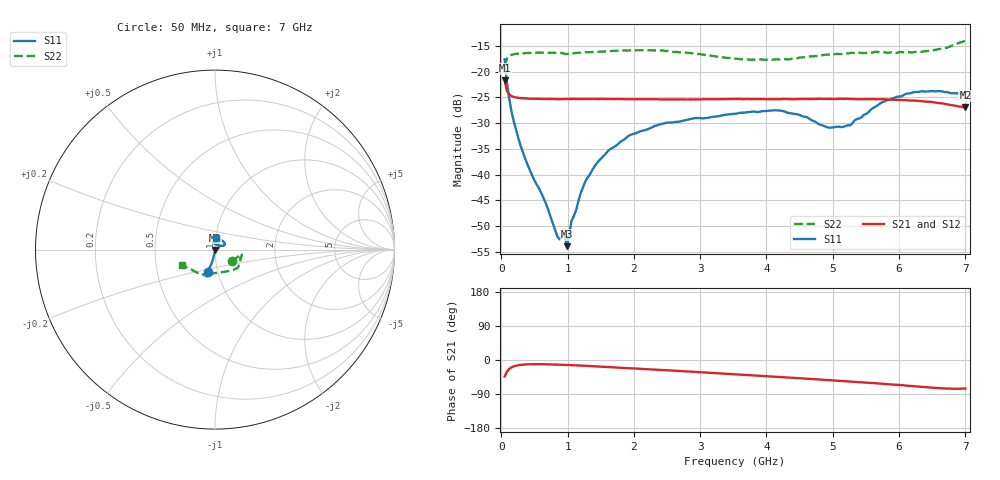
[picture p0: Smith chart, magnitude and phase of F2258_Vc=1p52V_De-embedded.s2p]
! Integrated Device Technology
! Corporate Headquarters
! 6024 Silver Creek Valley Road
! San Jose, CA 95138  USA
! Phone:  1-408-284-8200
! Toll Free:  1-800-223-1366
! Webpage:  http://www.idt.com/
! Timing and RF Division
! 515 Groton Road, Suite 102
! Westford, MA 01886-6024
! Device:  F2258
! Description: Voltage Variable RF Attenuator
! Frequency:  50.0 -  6000.00 MHz
! Package:  3x3 mm Thin QFN Plastic Package: 16 pin
! Ports:  2 RF, 2 DC
!  Pin  1  = NC
!  Pin  2  = NC
!  Pin  3  = RF2  = Port 2
!  Pin  4  = GND
!  Pin  5  = Vdd
!  Pin  6  = NC
!  Pin  7  = VCTRL
!  Pin  8  = NC
!  Pin  9  = GND
!  Pin 10  = RF1  = Port 1
!  Pin 11  = NC
!  Pin 12  = NC
!  Pin 13  = NC
!  Pin 14  = NC
!  Pin 15  = NC
!  Pin 16  = NC
! Vcntrl:  1.520 Volts
! Vdd:  +3.300 Volts
! Current:  1.161 mA
! Data:  The device was measured on a the F2258 evaluation board which has
!  individual transmission lines to the RF pins.  Data was collected
!  using a calibrated network analyzer.  The evaluation board was
!  de-embedded using a TRL calibration technique.
!  The reference plane is the edge of the package pin.
! Misc:  SN 10
!  Action Tracker AT0285
! Date Measured:  2014-12-10
! Date:  2016-01-13  MJV
! Note:
!  Integrated Device Technology supplies this data as a sample of measured
!  data at the package pin for this product.  Your particular data for this
!  product may vary.
!  Data was taken at 25 degrees C.
!  Integrated Device Technology reserves the right to change this data at anytime.
!Freq_(GHz)  S11M_(dB)  S11P_(deg)  S21M_(dB)  S21P_(deg)  S12M_(dB)  S12P_(deg)  S22M_(dB)  S22P_(deg)
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# GHz S dB R 50
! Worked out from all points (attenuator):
!   201 points, 50 MHz to 7 GHz, reference 50 ohm
!   highest |S21| = -21.70 dB at 50 MHz (marker M1); lowest = -26.9 dB at 7 GHz (marker M2)
!   lowest |S11| = -53.9 dB at 988.2 MHz (marker M3), VSWR 1.00, Z = 50.1 - j0.176 ohm
!   |S11| at or under -10 dB: start of sweep to end of sweep
!   |S22| runs from -18.9 to -14.0 dB; largest |S21 - S12| = 0.00055
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0.05  -17.62 -108.5  -21.70 -43.6  -21.68 -43.6  -18.89 -34.7
0.08475  -22.09 -103.7  -23.76 -30.8  -23.69 -30.7  -17.45 -17.1
0.15425  -27.76 -101.1  -24.75 -19.4  -24.71 -19.4  -16.75 -10.5
0.29325  -34.48 -98.7  -25.14 -12.8  -25.11 -12.8  -16.46 -9.0
0.6755  -45.66 -77.9  -25.30 -11.4  -25.28 -11.4  -16.30 -13.3
0.84925  -52.10 -35.2  -25.35 -12.2  -25.31 -12.2  -16.39 -16.4
0.9535  -51.45 -74.7  -25.34 -12.9  -25.31 -12.9  -16.58 -17.8
0.98825  -53.86 -60.1  -25.34 -13.1  -25.28 -13.1  -16.59 -18.8
1.05775  -49.03 -14.0  -25.31 -13.6  -25.30 -13.6  -16.46 -19.8
1.2315  -42.44 10.9  -25.31 -15.0  -25.28 -15.0  -16.28 -22.7
1.40525  -38.42 14.1  -25.30 -16.7  -25.27 -16.7  -16.17 -25.3
1.61375  -35.34 19.1  -25.33 -18.7  -25.28 -18.7  -16.04 -29.0
1.9265  -32.41 27.9  -25.37 -21.7  -25.33 -21.7  -15.89 -33.5
2.37825  -30.28 39.3  -25.40 -26.0  -25.37 -26.0  -15.91 -40.5
3.525  -28.20 87.5  -25.32 -37.7  -25.35 -37.7  -17.47 -68.1
4.1505  -27.50 103.4  -25.35 -44.4  -25.35 -44.4  -17.61 -88.9
4.7065  -29.57 93.5  -25.30 -50.4  -25.31 -50.4  -17.05 -100.5
4.94975  -30.89 76.2  -25.31 -53.1  -25.33 -53.1  -16.71 -103.1
5.2625  -30.43 48.0  -25.33 -56.7  -25.34 -56.7  -16.39 -105.4
5.85325  -25.45 25.7  -25.44 -64.2  -25.44 -64.2  -16.34 -108.9
6.33975  -23.78 32.0  -25.75 -71.0  -25.75 -71.0  -16.16 -120.6
7  -23.95 83.6  -26.95 -75.2  -27.04 -75.2  -13.96 -154.8
